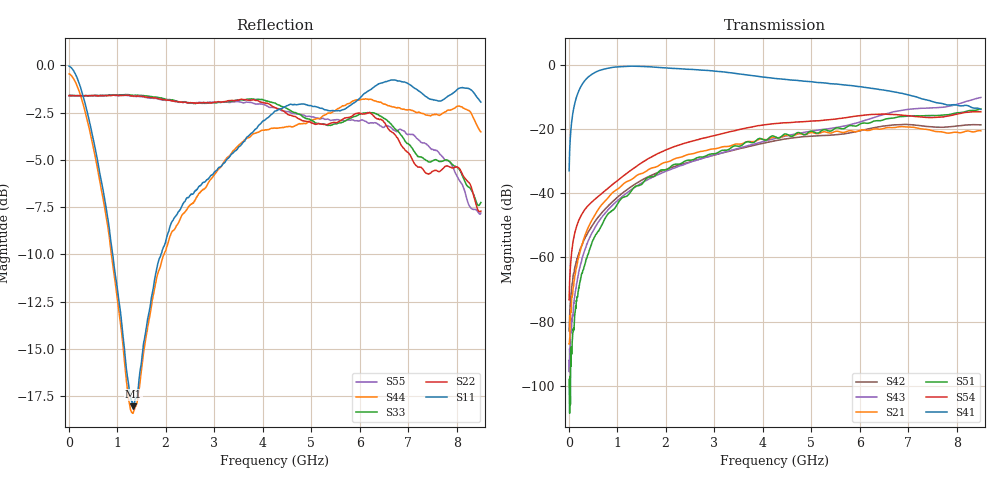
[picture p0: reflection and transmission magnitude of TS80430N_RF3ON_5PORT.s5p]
!Created with skrf (http://scikit-rf.org).
# GHz S RI R 50.0
!freq ReS11 ImS11 ReS12 ImS12 ReS13 ImS13
! ReS14 ImS14 ReS15 ImS15
! ReS21 ImS21 ReS22 ImS22 ReS23 ImS23
! ReS24 ImS24 ReS25 ImS25
! ReS31 ImS31 ReS32 ImS32 ReS33 ImS33
! ReS34 ImS34 ReS35 ImS35
! ReS41 ImS41 ReS42 ImS42 ReS43 ImS43
! ReS44 ImS44 ReS45 ImS45
! ReS51 ImS51 ReS52 ImS52 ReS53 ImS53
! ReS54 ImS54 ReS55 ImS55
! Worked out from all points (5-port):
!   1601 points, 10 MHz to 8.5 GHz, reference 50 ohm
!   strongest paths, dB at 10 MHz, 2.132 GHz, 4.255 GHz, 6.378 GHz, 8.5 GHz:
!     S41: -33.0, -1.0, -4.2, -7.5, -13.8
!     S54: -73.2, -25.7, -18.3, -15.3, -14.6
!     S51: -98.1, -31.3, -22.3, -17.3, -13.7
!     S21: -87.0, -29.6, -22.5, -19.9, -20.5
!     S43: -92.1, -32.4, -22.9, -15.9, -10.1
!     S42: -83.0, -31.9, -23.6, -19.3, -18.6
!   lowest |S11| = -18.0 dB at 1.337 GHz (marker M1), VSWR 1.29, Z = 39.2 + j2.88 ohm
!   |S11| at or under -10 dB: 907.8 MHz to 1.903 GHz (995.4 MHz wide, 70.8 % of centre)
